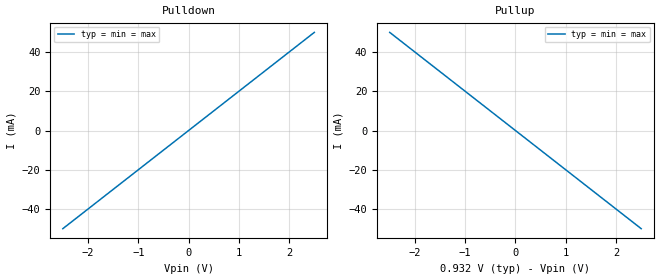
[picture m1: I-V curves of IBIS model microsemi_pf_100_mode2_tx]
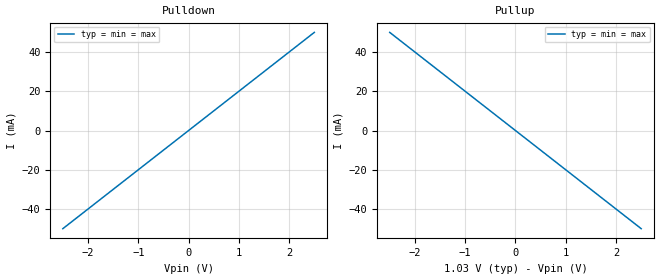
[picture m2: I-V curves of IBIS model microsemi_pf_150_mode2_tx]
|   Microsemi MPF300XT IBIS-AMI Model
[IBIS Ver]   6.0
[Disclaimer] THIS IBIS MODEL HAS BEEN CREATED BY THE SIGNAL
   INTEGRITY SOFTWARE SPICE WRAPPING PROCESS.
   THESE IBIS MODELS AREPROVIDED "AS IS" WITH NO
   WARRANTY WHATSOEVER AND SIGNAL INTEGRITY SOFTWARE
   SPECIFICALLY DISCLAIMS ANY IMPLIED WARRANTIES OF
   MERCHANTABILITY, FITNESS FOR A PARTICULAR PURPOSE,
   OR AGAINST INFRINGEMENT.
[File Name]  mpf300xt_ami.ibs
[Date]   Feb 16, 2018
[File Rev]   1.0
[Source]   Microsemi PolarFire MPF300XT AMI model provided by SiSoft
[Notes]   Revision 1.0
|   Initial Release
[Copyright]  Copyright 2018, Microsemi Corporation, All Rights Reserved.
|   COMPONENT: microsemi_pf_serdes
[Component] microsemi_pf_serdes
[Manufacturer]  Microsemi
[Package]
R_pkg   0.001m  NA NA
L_pkg   0.000nH NA NA
C_pkg   0.000pF NA NA
[Pin] signal_name   model_name   R_pin L_pin C_pin
3   microsemi_pf_100_m2_tx_p   microsemi_pf_100_mode2_tx  NA   NA   NA
4   microsemi_pf_100_m2_tx_n   microsemi_pf_100_mode2_tx  NA   NA   NA
5   microsemi_pf_150_m2_tx_p   microsemi_pf_150_mode2_tx  NA   NA   NA
6   microsemi_pf_150_m2_tx_n   microsemi_pf_150_mode2_tx  NA   NA   NA
[Diff Pin] inv_pin  vdiff tdelay_typ tdelay_min tdelay_max
3   4   0.050 na   na   na
5   6   0.050 na   na   na
| Models and submodels in the file (2): microsemi_pf_100_mode2_tx (Output), microsemi_pf_150_mode2_tx (Output)
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|   MODEL microsemi_pf_100_mode2_tx
[Model] microsemi_pf_100_mode2_tx
|SiSoft ModelSignature3 41179604a350c70a0706564fda80a1c02d77ce3dc9b9310286028757333490fb Certified
Model_type Output
C_comp 0.3p 0.2p 0.5p
Vmeas = 0.575
Vref = 0.575
Rref = 50
Cref = 1pf
[Model Spec]
[Algorithmic Model]
Executable Linux_gcc4.4.7_64   microsemi_PF_tx_glnxa64.so microsemi_pf_100_mode2_tx.ami
Executable Windows_cl18.00.40629_64 microsemi_PF_tx_win64.dll  microsemi_pf_100_mode2_tx.ami
[End Algorithmic Model]
[Temperature Range]  40 100 -40
[Voltage Range] 0.932 0.870 0.992
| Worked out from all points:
|   slope of the pulldown table from 0 to 0.14 V, typ, clamps not added: 50 ohm
|   slope of the pullup table from 0 to 0.14 V, typ, clamps not added: 50 ohm
[Pulldown]
-2.5V     -50mA      -50mA      -50mA
0V        0A         0A         0A
2.5V      50mA       50mA       50mA
[Pullup]
-2.5V     50mA       50mA       50mA
0V        0A         0A         0A
2.5V      -50mA      -50mA      -50mA
[Ramp]
dV/dt_r 0.2796/15p   0.2610/23.5p   0.2976/13p
dV/dt_f 0.2796/15p   0.2610/23.5p   0.2976/13p
|   MODEL microsemi_pf_150_mode2_tx
[Model] microsemi_pf_150_mode2_tx
|SiSoft ModelSignature3 27583a96385ed2163102d7608887ab210514215b35cefaae48b5f7d6e5b35c19 Certified
Model_type Output
C_comp 0.3p 0.2p 0.5p
Vmeas = 0.575
Vref = 0.575
Rref = 50
Cref = 1pf
[Model Spec]
[Algorithmic Model]
Executable Linux_gcc4.4.7_64   microsemi_PF_tx_glnxa64.so microsemi_pf_150_mode2_tx.ami
Executable Windows_cl18.00.40629_64 microsemi_PF_tx_win64.dll  microsemi_pf_150_mode2_tx.ami
[End Algorithmic Model]
[Temperature Range]  40 100 -40
[Voltage Range] 1.032 0.962 1.102
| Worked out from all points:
|   slope of the pulldown table from 0 to 0.155 V, typ, clamps not added: 50 ohm
|   slope of the pullup table from 0 to 0.155 V, typ, clamps not added: 50 ohm
[Pulldown]
-2.5V     -50mA      -50mA      -50mA
0V        0A         0A         0A
2.5V      50mA       50mA       50mA
[Pullup]
-2.5V     50mA       50mA       50mA
0V        0A         0A         0A
2.5V      -50mA      -50mA      -50mA
[Ramp]
dV/dt_r 0.3096/17p   0.2886/24p   0.3306/14p
dV/dt_f 0.3096/17p   0.2886/24p   0.3306/14p
